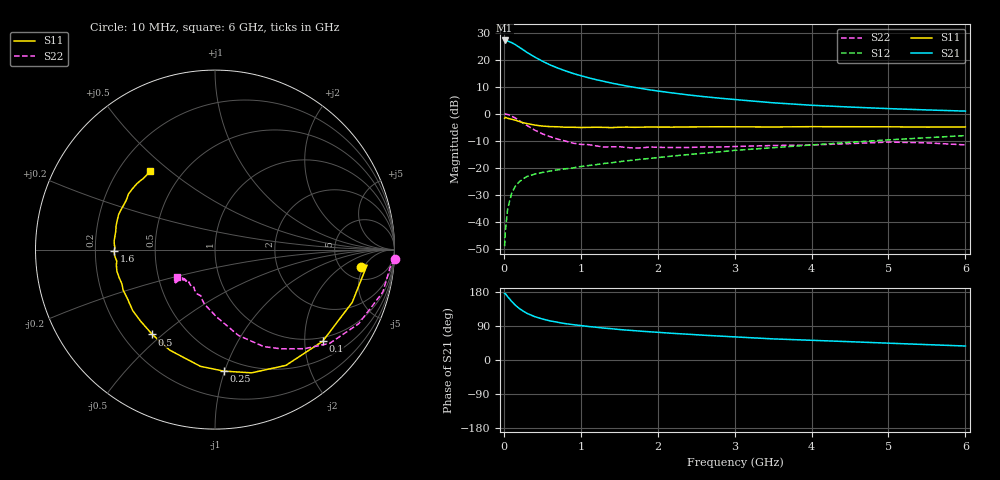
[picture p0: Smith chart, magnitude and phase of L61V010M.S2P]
!  INFINEON TECHNOLOGIES Small Signal Semiconductors
! BFR380L3 , Si-NPN RF-Transistor in TSLP-3-1
!  Vce=1 V,  Ic=10 mA
! Common Emitter S-Parameters:  07. March 2005
#  GHz  S  MA  R  50
! f  S11  S21  S12  S22
! GHz  Mag  Ang  Mag  Ang  Mag  Ang  Mag  Ang
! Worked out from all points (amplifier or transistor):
!   36 points, 10 MHz to 6 GHz, reference 50 ohm
!   highest |S21| = 27.1 dB at 10 MHz (marker M1)
!   |S21| within 3 dB of that: start of sweep to 226.9 MHz
!   unconditionally stable (mu >= 1): 2.027 GHz to 4.963 GHz
!   at 250 MHz: K = 0.27, MSG = 23.9 dB, |S12| = -24.2 dB
!   at 1.4 GHz: K = 0.90, MSG = 14.8 dB, |S12| = -18.2 dB
!   at 6 GHz: K = 0.98, MSG = 4.5 dB, |S12| = -8.1 dB
!   S11 on the Smith chart (normalised r, x): 10 MHz: 7.53, -4.42; 100 MHz: 0.90, -2.43; 250 MHz: 0.40, -0.99; 500 MHz: 0.32, -0.46; 1.6 GHz: 0.28, -0.01; 6 GHz: 0.33, +0.43
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0.01  0.8207 -6.7  22.67 175.6  0.0035 81.2  1.002 -2.9
0.02  0.8516 -5.8  22.65 175.0  0.0068 88.6  0.9805 -5.9
0.05  0.8192 -21.0  22.13 167.0  0.0172 80.8  0.9646 -14.2
0.1  0.7878 -40.4  20.7 155.1  0.0331 71.8  0.9007 -27.3
0.15  0.7564 -58.5  18.95 144.6  0.0455 62.8  0.8257 -39.2
0.2  0.7161 -73.5  17.01 136.0  0.0545 57.5  0.7442 -47.9
0.25  0.6786 -85.9  15.27 129.3  0.0619 52.9  0.6627 -56.5
0.3  0.6554 -97.1  13.66 123.3  0.0682 49.9  0.6049 -63.3
0.4  0.6144 -114.2  11.21 114.5  0.0756 46.2  0.496 -74.7
0.5  0.5879 -126.5  9.393 108.3  0.0812 44.5  0.423 -81.8
0.6  0.5749 -136.5  8 103.3  0.0861 43.8  0.3747 -88.7
0.7  0.5704 -143.6  6.996 99.5  0.0909 44.6  0.3367 -94.9
0.9  0.5592 -156.3  5.548 93.3  0.0987 46.1  0.2832 -105.3
1.1  0.5561 -163.7  4.616 88.4  0.1091 47.7  0.2662 -111.8
1.4  0.5513 -173.3  3.678 82.6  0.1229 50.2  0.2428 -119.7
1.6  0.563 -179.0  3.242 78.8  0.1337 51.6  0.2354 -127.6
2.2  0.5622 169.6  2.407 70.3  0.1641 55.1  0.2354 -132.3
2.8  0.5713 160.1  1.935 63.2  0.1955 57.3  0.24 -138.8
3.5  0.5656 151.1  1.587 55.7  0.2334 57.3  0.2567 -139.3
4.5  0.5715 144.0  1.323 48.3  0.294 57.7  0.2783 -139.9
5.5  0.5627 135.1  1.17 40.6  0.3578 55.3  0.2872 -141.1
6  0.5659 129.6  1.113 36.9  0.3915 53.5  0.2634 -144.3
